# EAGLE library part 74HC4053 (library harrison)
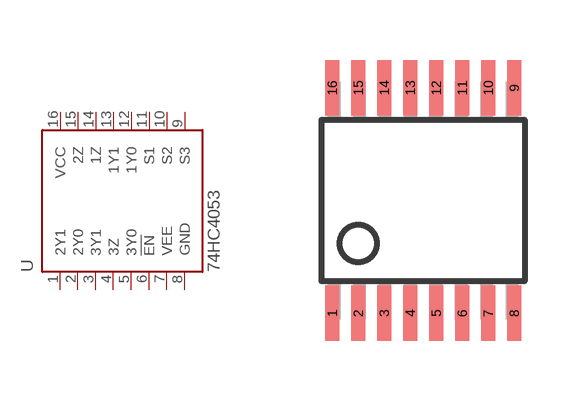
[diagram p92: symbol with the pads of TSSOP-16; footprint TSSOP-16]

Designator prefix U

## 74HC4053_TSSOP-16  [TSSOP-16]
1  2Y1
2  2Y0
3  3Y1
4  3Z
5  3Y0
6  !EN!  in
7  VEE  pwr
8  GND  pwr
9  S3  in
10  S2  in
11  S1  in
12  1Y0
13  1Y1
14  1Z
15  2Z
16  VCC  pwr

## Footprint TSSOP-16 (pad centres in mm)
smd 0.348 x 1.397: 1 -2.273,-2.814; 2 -1.623,-2.815; 3 -0.973,-2.815; 4 -0.323,-2.815; 5 0.327,-2.815; 6 0.977,-2.815; 7 1.627,-2.815; 8 2.277,-2.815; 9 2.277,2.825; 10 1.627,2.825; 11 0.977,2.825; 12 0.327,2.825; 13 -0.323,2.825; 14 -0.973,2.825; 15 -1.623,2.825; 16 -2.273,2.825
